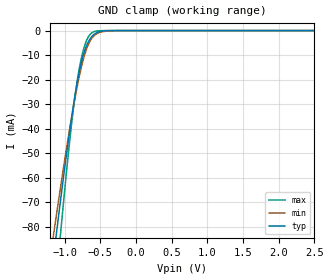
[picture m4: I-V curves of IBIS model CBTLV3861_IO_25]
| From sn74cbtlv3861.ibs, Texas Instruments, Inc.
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[Model]   CBTLV3861_IO_25
Model_type  Terminator
| variable   typ   min   max
C_comp   4.10pF   3.63pF   4.57pF
| C_tri-state   4.10pF   3.63pF   4.57pF
[Temperature Range]   40   100   -40
| Ambient temperature   25   85   -40
[Voltage range]   2.5   2.3   2.7
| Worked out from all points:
|   GND clamp passes 1 mA (typ) near -0.56 V on its own axis
[GND Clamp]
| CBTLV3861_IO_25
|   Voltage   I(typ)   I(min)   I(max)
-2.5V     -461.9mA   -388.1mA   -585.6mA
-1.165V   -95.06mA   -85.52mA   -117.6mA
-1.14V    -89.01mA   -80.47mA   -109.5mA
-1.1V     -79.47mA   -72.5mA    -96.72mA
-1.06V    -70.11mA   -64.65mA   -84.12mA
-1.04V    -65.5mA    -60.79mA   -77.91mA
-905mV    -36.3mA    -36.04mA   -38.92mA
-815mV    -20.09mA   -21.68mA   -19.16mA
-720mV    -8.383mA   -10.04mA   -6.3mA
-605mV    -2.037mA   -2.684mA   -684.9uA
-275mV    -2.887uA   -26.87uA   -33.07nA
2.5V      7.048nA    100.3nA    45.48pA
